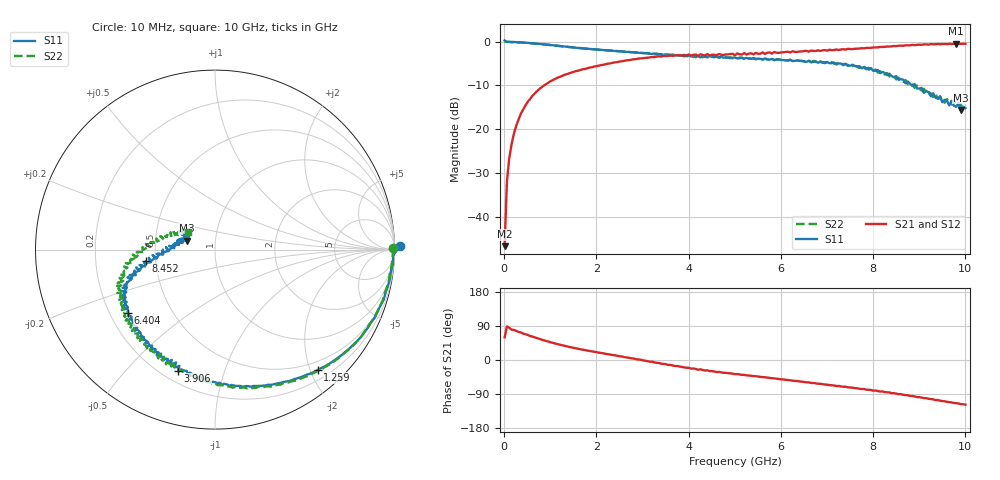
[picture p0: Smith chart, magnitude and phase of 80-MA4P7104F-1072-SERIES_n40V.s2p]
!Agilent Technologies,E8364C,MY48140145,A.09.42.15
!Agilent E8364C: A.09.42.15
!Date: Wednesday, December 02, 2020 07:37:46
!Correction: S11(Full 2 Port(1,2))
!S21(Full 2 Port(1,2))
!S12(Full 2 Port(1,2))
!S22(Full 2 Port(1,2))
!S2P File: Measurements: S11, S21, S12, S22:
# Hz S  dB  R 50
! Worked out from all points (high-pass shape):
!   201 points, 10 MHz to 10 GHz, reference 50 ohm
!   highest |S21| = -0.50 dB at 9.8 GHz (marker M1); lowest = -46.7 dB at 10 MHz (marker M2)
!   |S21| within 3 dB of the highest: 3.284 GHz to end of sweep
!   lowest |S11| = -15.6 dB at 9.9 GHz (marker M3), VSWR 1.40, Z = 36.2 + j3.76 ohm
!   |S11| at or under -10 dB: 8.834156 GHz to 8.871143 GHz (36.99 MHz wide, 0.418 % of centre); 8.914 GHz to end of sweep
!   |S22| runs from -15.5 to -0.1 dB; largest |S21 - S12| = 0.025
!   S11 on the Smith chart (normalised r, x): 10 MHz: -47, +34; 1.259 GHz: 0.35, -2.12; 3.906 GHz: 0.26, -0.71; 6.404 GHz: 0.27, -0.30; 8.452 GHz: 0.44, -0.07; 10 GHz: 0.72, +0.10
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1e7  0.24 1.1  -46.75 59.8  -41.76 92.5  -0.05 0.4
5.995e7  -0.06 -1.9  -32.02 88.7  -31.87 89.6  -0.10 -2.8
1.099e8  -0.06 -4.8  -26.70 85.0  -26.65 83.9  -0.10 -5.2
1.5985e8  -0.11 -7.3  -23.53 80.0  -23.44 80.1  -0.15 -7.5
2.5975e8  -0.14 -12.1  -19.32 76.7  -19.35 76.1  -0.17 -12.4
6.094e8  -0.38 -26.9  -12.43 61.8  -12.43 62.1  -0.42 -27.6
1.25875e9  -1.09 -49.5  -7.83 38.8  -7.82 38.8  -1.11 -51.3
1.7083e9  -1.56 -61.6  -6.33 27.2  -6.33 27.3  -1.55 -64.1
3.35665e9  -2.86 -97.0  -3.39 -7.8  -3.38 -8.6  -2.93 -100.0
3.9061e9  -3.03 -106.9  -3.19 -19.6  -3.13 -19.2  -3.40 -110.3
5.005e9  -3.66 -122.6  -3.14 -37.5  -3.08 -36.6  -3.63 -129.5
6.4036e9  -4.43 -143.9  -2.28 -56.4  -2.26 -56.5  -4.37 -149.9
6.7033e9  -4.66 -148.8  -2.14 -60.8  -2.15 -60.6  -4.41 -154.7
7.9021e9  -6.39 -163.2  -1.44 -78.7  -1.48 -78.6  -5.99 -171.4
8.35165e9  -7.34 -168.5  -1.15 -85.6  -1.11 -86.6  -7.95 -178.0
8.45155e9  -8.14 -170.5  -1.02 -87.5  -1.09 -88.1  -7.89 -179.7
9.2008e9  -11.64 -178.0  -0.70 -102.5  -0.63 -101.8  -11.53 158.7
9.75025e9  -14.66 168.5  -0.55 -113.4  -0.53 -112.7  -13.53 149.1
9.8002e9  -14.93 159.6  -0.50 -113.8  -0.54 -114.1  -14.77 153.3
9.85015e9  -14.02 162.3  -0.57 -114.9  -0.51 -114.8  -14.50 144.3
9.9001e9  -15.61 162.3  -0.52 -116.3  -0.51 -115.9  -14.26 150.5
1e10  -15.21 156.2  -0.51 -117.9  -0.51 -118.0  -15.00 147.1
